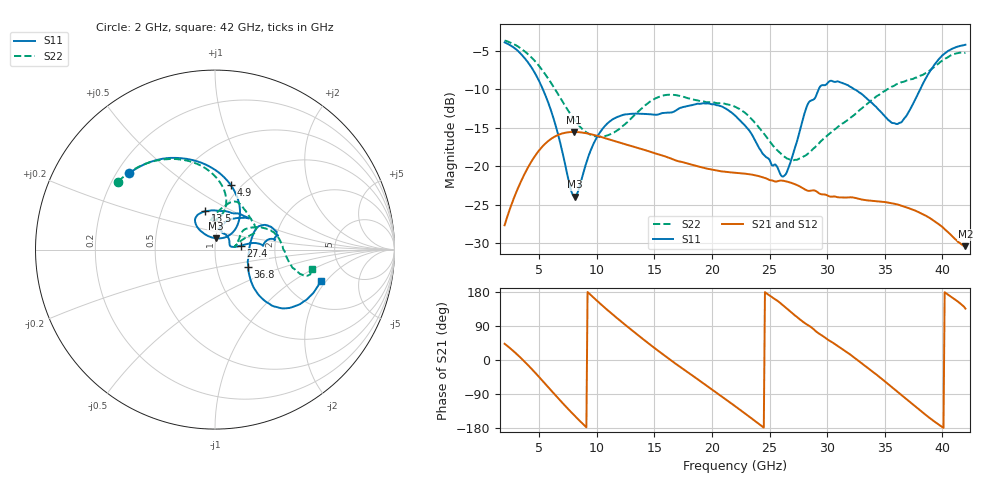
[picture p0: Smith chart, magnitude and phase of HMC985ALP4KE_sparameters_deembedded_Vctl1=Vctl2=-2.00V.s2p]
!s2p File: Measurements: S11, S21, S12, S22
# GHz S dB R 50.0
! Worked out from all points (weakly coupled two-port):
!   401 points, 2 GHz to 42 GHz, reference 50 ohm
!   highest |S21| = -15.52 dB at 8 GHz (marker M1); lowest = -30.4 dB at 42 GHz (marker M2)
!   lowest |S11| = -24.0 dB at 8.1 GHz (marker M3), VSWR 1.14, Z = 50 + j6.35 ohm
!   |S11| at or under -10 dB: 5.329 GHz to 29.26 GHz (23.93 GHz wide, 138 % of centre); 32.39 GHz to 38.06 GHz (5.675 GHz wide, 16.1 % of centre)
!   |S22| runs from -19.2 to -3.6 dB; largest |S21 - S12| = 0.00015
!   S11 on the Smith chart (normalised r, x): 2 GHz: 0.25, +0.36; 4.9 GHz: 0.90, +0.75; 13.5 GHz: 0.82, +0.37; 27.4 GHz: 1.34, +0.06; 36.8 GHz: 1.42, -0.29; 42 GHz: 3.15, -1.78
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2  -3.87 138.4  -27.68 42.8  -27.68 42.8  -3.62 144.9
3.4  -5.35 109.6  -22.04 5.7  -22.04 5.7  -4.65 121.3
4.9  -8.62 76.4  -18.11 -41.7  -18.12 -41.7  -6.77 97.1
6.1  -13.07 52.1  -16.36 -82.4  -16.37 -82.4  -9.31 82.0
8  -23.90 79.1  -15.52 -144.6  -15.53 -144.6  -13.83 78.1
8.1  -23.96 86.0  -15.53 -147.7  -15.53 -147.7  -14.03 78.8
8.7  -21.60 116.1  -15.60 -165.9  -15.60 -165.9  -15.09 83.9
10.6  -14.94 126.9  -16.28 140.6  -16.29 140.6  -16.11 98.8
13.5  -13.14 104.4  -17.59 67.6  -17.59 67.6  -13.02 83.1
15.4  -13.23 80.1  -18.47 22.7  -18.48 22.7  -10.96 70.1
18.9  -11.87 44.2  -20.05 -53.8  -20.06 -53.8  -11.48 44.6
22  -13.38 55.1  -20.83 -121.6  -20.84 -121.6  -12.25 23.3
24.5  -18.50 78.3  -21.46 -178.5  -21.47 -178.5  -15.73 19.7
26.1  -21.33 18.5  -21.86 145.9  -21.87 145.9  -18.53 11.4
27.4  -16.66 8.7  -22.46 112.8  -22.46 112.8  -19.16 8.3
28.7  -11.38 4.6  -23.14 84.5  -23.15 84.4  -17.85 16.2
31.1  -9.05 17.1  -24.05 33.3  -24.05 33.3  -14.68 33.8
33.3  -10.97 27.9  -24.40 -15.4  -24.41 -15.4  -12.12 29.8
35.4  -14.07 8.1  -24.75 -66.1  -24.75 -66.1  -9.84 19.9
36.8  -13.60 -27.9  -25.30 -101.3  -25.30 -101.3  -8.90 10.8
39.7  -6.04 -41.0  -27.55 -170.7  -27.56 -170.8  -6.59 -15.1
42  -4.18 -16.5  -30.40 135.6  -30.41 135.8  -5.22 -11.1
